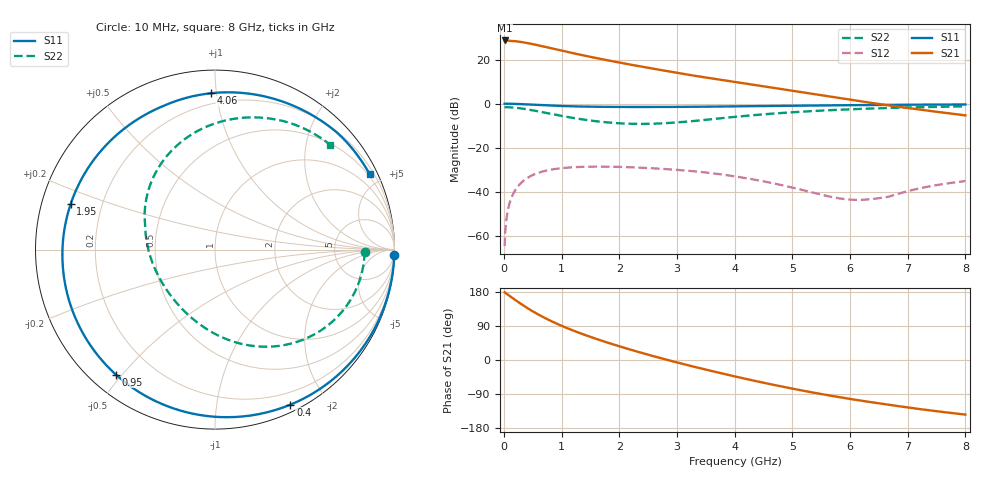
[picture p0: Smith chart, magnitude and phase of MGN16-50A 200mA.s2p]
! Port[1] = GATE
! Port[2] = DRAIN
! [Type]  S-parameter s2p file touchstone ver. 1.0
! [Object]  MGN16-50A
! [Bias]  200 mA
! [Version]  1.0
! [Date]  Thu May 28 11:04:55 2026
! [Source]  This file was created in JSC "ICC Milandr".
! [Disclaimer] Property of JSC "ICC Milandr". Unauthorized reproduction and/or distribution is strictly prohibited.
!  The file and the data are provided "AS IS" and with all faults and disclaim all warranties, express and implied, including
!  without limitation any implied warranties of merchantability, fitness for a particular purpose.
!  JSC "ICC Milandr" assumes no liability for:
!  1) the accuracy of the data provided;
!  2) the proper functioning of this data;
!  3) infringement of patents, copyrights or intellectual property rights resulting from the use of this data.
!  JSC "ICC Milandr" reserves the right to make changes to the products and the data without prior notice.
!  Please, be aware that your receipt and use of the file provided shall serve as acceptance of these terms and conditions.
!  If you do not accept these terms, you should return or destroy this file and any other accompanying information immediately.
# hz S ma R 12.5
! 2 Port Network Data from SP1.SP block
! freq  magS11  angS11  magS21  angS21  magS12  angS12  magS22  angS22
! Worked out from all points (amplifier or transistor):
!   800 points, 10 MHz to 8 GHz, reference 12.5 ohm
!   highest |S21| = 28.6 dB at 10 MHz (marker M1)
!   |S21| within 3 dB of that: start of sweep to 730.4 MHz
!   unconditionally stable (mu >= 1): 4.124 GHz to 7.987 GHz
!   at 1.34 GHz: K = 0.20, MSG = 25.4 dB, |S12| = -28.6 dB
!   at 4.01 GHz: K = 0.94, MSG = 21.4 dB, |S12| = -33.0 dB
!   at 8 GHz: K = 0.99, MSG = 14.9 dB, |S12| = -35.1 dB
!   S11 on the Smith chart (normalised r, x): 10 MHz: 2, -68; 400 MHz: 0.07, -1.60; 950 MHz: 0.07, -0.48; 1.95 GHz: 0.09, +0.15; 4.06 GHz: 0.13, +0.96; 8 GHz: 0.41, +4.27
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1e7  0.9991 -1.7  27.04 178.7  0.0005904 81.8  0.8334 -0.9
4e7  0.9987 -6.8  26.93 175.4  0.002333 83.8  0.8327 -3.9
9e7  0.9967 -15.3  26.74 169.9  0.005212 79.5  0.8284 -8.8
1.8e8  0.9897 -30.2  26.15 160.0  0.0102 70.4  0.8127 -17.5
2.9e8  0.9766 -47.7  25.04 148.4  0.01574 59.5  0.7824 -27.5
4e8  0.9607 -64.1  23.66 137.5  0.02054 49.2  0.744 -37.0
5.1e8  0.944 -79.2  22.16 127.4  0.02454 39.6  0.7017 -45.7
6.4e8  0.925 -95.5  20.36 116.3  0.0283 29.2  0.651 -55.2
7.9e8  0.9057 -112.4  18.37 104.7  0.03155 18.3  0.5956 -65.1
9.5e8  0.8887 -128.4  16.46 93.5  0.034 7.8  0.5426 -74.9
1.14e9  0.8732 -145.1  14.47 81.3  0.03587 -3.5  0.4892 -85.6
1.35e9  0.8608 -161.2  12.61 69.0  0.03702 -14.8  0.4417 -96.9
1.63e9  0.85 -179.6  10.6 54.1  0.0375 -28.5  0.3951 -111.5
1.95e9  0.8433 162.5  8.779 38.4  0.03706 -42.9  0.3622 -128.3
2.31e9  0.8405 145.5  7.186 22.1  0.03572 -57.9  0.3479 -147.4
2.68e9  0.8416 130.7  5.901 6.4  0.03371 -72.3  0.3549 -166.8
3.27e9  0.8495 111.4  4.358 -16.8  0.02961 -94.0  0.4019 164.8
4.01e9  0.87 92.7  3.1 -43.6  0.02244 -110.9  0.5036 136.7
4.06e9  0.8714 91.6  3.03 -45.3  0.02192 -111.8  0.5108 134.9
5.34e9  0.9067 65.4  1.668 -85.4  0.009763 -118.4  0.6784 95.9
6.67e9  0.9417 44.0  0.9117 -118.0  0.007788 -66.5  0.7986 65.4
8e9  0.9587 26.1  0.5427 -144.1  0.01764 -61.4  0.8672 42.4
